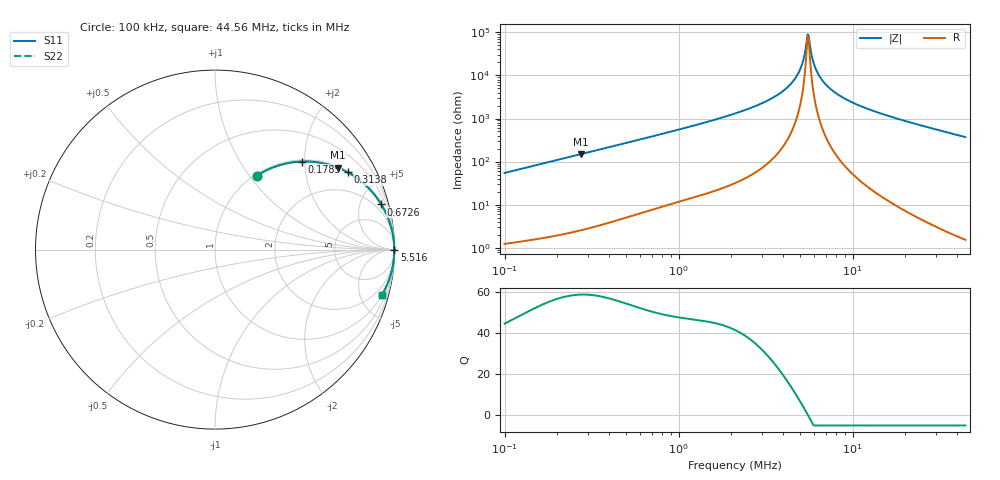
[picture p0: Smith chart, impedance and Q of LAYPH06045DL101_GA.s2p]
! LAYPH06045DL101_GA  S-PARAMETER MODEL  ( General Type )
! Model Generated by TAIYO YUDEN Corporation (http://www.ty-top.com)
! Version 2.0
! TAIYO YUDEN Control No. 180914NI43SB-FBB
! Copyright(c) 2018 TAIYO YUDEN CO.,LTD. All Rights Reserved.
! Product Description (link to TY-COMPAS)
! https://ds.yuden.co.jp/TYCOMPAS/or/detail?pn=LAYPH06045DL101MGA&u=M
! Products Name : Inductors
! Characteristics :
!  Inductance : 100 uH , SRF(min) : -Hz , DC Resistance(max) : 0.384 Ohm
!  Rated Current : Saturation :0.55 A , Temp Rise : 0.56 A (25 degC)
!  Case Size : 6.3 x 6.0 / 0.248 x 0.236 [mm/inch] , Thickness : 4.5 / 0.177 [mm/inch]
!  (Conditions: Temperature = 25 degC , DC Bias Current/Voltage = 0A / 0V)
! External Node Assignments :
!  1  o---GGG---o  2
! GND o---------o GND
! Frequency Range : 0.1MHz  -  44.556096MHz  [ 402 STEP ]
# MHz S RI R 50
! Freq[MHz].  S11 Real  S11 Imag  S21 Real  S21 Imag  S12 Real  S12 Imag  S22 Real  S22 Imag
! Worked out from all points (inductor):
!   401 points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, 100 kHz to 44.56 MHz, reference 50 ohm
!   read as one part in series: L = 86.5 uH near 103.1 kHz
!   highest Q = 58.6 at 273.6 kHz (marker M1), where L = 86.3 uH
!   self-resonance near 5.516 MHz
!   S11 on the Smith chart (normalised r, x): 100 kHz: 1.02, +1.09; 178.5 kHz: 1.04, +1.94; 313.8 kHz: 1.06, +3.40; 672.6 kHz: 1.14, +7.32; 5.516 MHz: open; 44.56 MHz: 1.03, -7.41
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0.1  0.2342 0.4124  0.7658 -0.4124  0.7658 -0.4124  0.2342 0.4124
0.178503  0.4847 0.4908  0.5153 -0.4908  0.5153 -0.4908  0.4847 0.4908
0.273571  0.6846 0.4562  0.3154 -0.4562  0.3154 -0.4562  0.6846 0.4562
0.277774  0.691 0.4536  0.309 -0.4536  0.309 -0.4536  0.691 0.4536
0.313812  0.7397 0.4303  0.2603 -0.4303  0.2603 -0.4303  0.7397 0.4303
0.672641  0.9264 0.2515  0.0736 -0.2515  0.0736 -0.2515  0.9264 0.2515
0.771585  0.9427 0.2226  0.0573 -0.2226  0.0573 -0.2226  0.9427 0.2226
2.143265  0.9926 0.0743  0.00738 -0.0743  0.00738 -0.0743  0.9926 0.0743
3.284727  0.9973 0.0373  0.00271 -0.0373  0.00271 -0.0373  0.9973 0.0373
4.322153  0.9986 0.0172  0.00143 -0.0172  0.00143 -0.0172  0.9986 0.0172
4.957932  0.9989 0.00771  0.00113 -0.00771  0.00113 -0.00771  0.9989 0.00771
5.19  0.9989 0.00458  0.00108 -0.00458  0.00108 -0.00458  0.9989 0.00458
5.432931  0.999 0.00146  0.00104 -0.00146  0.00104 -0.00146  0.999 0.00146
5.516409  0.999 0.000421  0.00104 -0.000421  0.00104 -0.000421  0.999 0.000421
5.687232  0.999 -0.00166  0.00103 0.00166  0.00103 0.00166  0.999 -0.00166
5.863346  0.999 -0.00374  0.00103 0.00374  0.00103 0.00374  0.999 -0.00374
6.137794  0.9989 -0.00686  0.00105 0.00686  0.00105 0.00686  0.9989 -0.00686
6.425089  0.9989 -0.01  0.0011 0.01  0.0011 0.01  0.9989 -0.01
7.715185  0.9985 -0.0228  0.00148 0.0228  0.00148 0.0228  0.9985 -0.0228
10.30788  0.9971 -0.0449  0.00295 0.0449  0.00295 0.0449  0.9971 -0.0449
16.28686  0.9913 -0.0877  0.00868 0.0877  0.00868 0.0877  0.9913 -0.0877
44.5561  0.9312 -0.2511  0.0688 0.2511  0.0688 0.2511  0.9312 -0.2511
